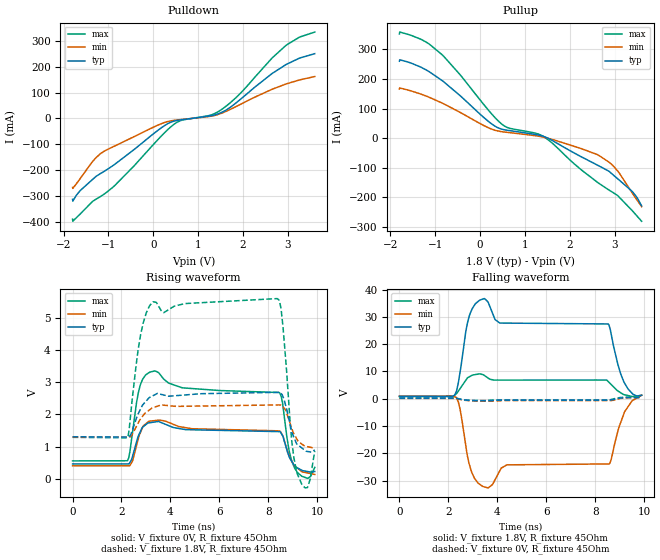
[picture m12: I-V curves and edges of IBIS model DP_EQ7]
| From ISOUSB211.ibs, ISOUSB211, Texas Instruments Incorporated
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[Model]   DP_EQ7
Model_type   Output
Polarity   Non-Inverting
Vmeas = 0.2
Vref = 0
Cref = 15pF
Rref = 45
|   typ   min   max
C_comp   5pF   3pF   8pF
[Voltage Range]   1.8   1.71   1.89
[Temperature Range]   27   150   -40
[Pullup Reference]   1.8   1.71   1.89
[Pulldown Reference]   0   0   0
[Power Clamp Reference]   1.8   1.71   1.89
[GND Clamp Reference]   0   0   0
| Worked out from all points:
|   slope of the pulldown table from 0 to 0.27 V, typ, clamps not added: 7.95 ohm
|   slope of the pullup table from 0 to 0.27 V, typ, clamps not added: 7.94 ohm
|   falling waveform, V_fixture 1.8V, R_fixture 45Ohm: 20-80 % time 71.7ps typ, 40.9ps min, 34.1ps max; typ from 0.895 V to 1.3 V
|   rising waveform, V_fixture 0V, R_fixture 45Ohm: 20-80 % time 286ps typ, 394ps min, 61.1ps max; typ from 0.46 V to 0.225 V
|   rising waveform, V_fixture 1.8V, R_fixture 45Ohm: 20-80 % time 252ps typ, 310ps min, 40.9ps max; typ from 1.3 V to 0.895 V
|   falling waveform, V_fixture 0V, R_fixture 45Ohm: 20-80 % time 184ps typ, 235ps min, 124ps max; typ from 0.225 V to 0.46 V
[Pulldown]
|   Voltage   I(typ)   I(min)   I(max)
-1.8V     -312.3mA   -266.2mA   -388.8mA
-1.795V   -319mA     -269.8mA   -396.8mA
-1.633V   -278.9mA   -232.8mA   -369.2mA
-1.179V   -212.7mA   -136mA     -301.6mA
-865.8mV  -177.8mA   -106.8mA   -260mA
73.8mV    -49.63mA   -27.98mA   -87.09mA
538.2mV   -7.266mA   -5.626mA   -13.71mA
1.294V    10.85mA    9.019mA    13.98mA
1.521V    23.18mA    20.15mA    34.45mA
1.899V    67.71mA    50.57mA    89.7mA
2.947V    206.8mA    132.3mA    280.4mA
3.6V      250.2mA    161.9mA    333.6mA
[Pullup]
|   Voltage   I(typ)   I(min)   I(max)
-1.8V     259.8mA    166.3mA    352.1mA
-1.795V   264.8mA    169.7mA    358.5mA
-1.325V   240.1mA    149.1mA    334.3mA
-849.6mV  194.9mA    118.9mA    282mA
381.6mV   36.3mA     24.84mA    61.51mA
613.8mV   26.64mA    19.55mA    35.63mA
1.402V    6.733mA    3.773mA    6.537mA
2.612V    -90.76mA   -55.24mA   -148.5mA
2.876V    -112.3mA   -81.28mA   -175.5mA
3.065V    -136.9mA   -110.7mA   -193.6mA
3.4V      -181.3mA   -187.3mA   -246.2mA
3.6V      -228.6mA   -231.2mA   -280.5mA
[Ramp]
R_load = 45
|   typ   min   max
dV/dt_r   0.140808/2.64432e-10   0.160407/3.48337e-10   0.120509/6.22032e-11
dV/dt_f   0.243789/4.77414e-11  0.210518/7.09993e-11   0.256824/2.36305e-09
[Falling Waveform]
V_fixture = 1.8V
V_fixture_min = 1.71V
V_fixture_max = 1.89V
R_fixture = 45Ohm
C_fixture = 0F
|   Time   V(typ)   V(min)   V(max)
0s        895mV      947.6mV    856.5mV
2.257ns   1.255V     713.3mV    1.343V
2.476ns   9.653V     -3.712V    3.69V
2.855ns   30.31V     -23.96V    8.039V
3.46ns    36.69V     -32.24V    8.615V
3.806ns   31.3V      -31.38V    6.957V
4.105ns   27.73V     -26.32V    6.853V
8.533ns   27.4V      -23.87V    6.319V
9.166ns   6.353V     -5.673V    1.535V
9.9ns     1.301V     1.298V     1.285V
[Rising Waveform]
V_fixture = 0V
V_fixture_min = 0V
V_fixture_max = 0V
R_fixture = 45Ohm
C_fixture = 0F
|   Time   V(typ)   V(min)   V(max)
0s        459.5mV    400.3mV    553.4mV
2.245ns   459.5mV    402.3mV    558.4mV
2.761ns   1.448V     1.411V     2.887V
3.359ns   1.76V      1.803V     3.343V
4.462ns   1.544V     1.604V     2.826V
8.444ns   1.462V     1.486V     2.675V
8.85ns    692mV      709.9mV    876.5mV
9.059ns   419.8mV    415mV      358.5mV
9.607ns   223.6mV    178.4mV    12.81mV
9.9ns     224.9mV    133mV      352.5mV
[Rising Waveform]
V_fixture = 1.8V
V_fixture_min = 1.71V
V_fixture_max = 1.89V
R_fixture = 45Ohm
C_fixture = 0F
|   Time   V(typ)   V(min)   V(max)
0s        1.301V     1.298V     1.285V
2.245ns   1.292V     1.295V     1.27V
2.776ns   2.156V     1.853V     4.442V
3.277ns   2.572V     2.202V     5.484V
8.356ns   2.679V     2.29V      5.587V
8.523ns   2.645V     2.285V     5.271V
8.96ns    1.458V     1.563V     1.169V
9.15ns    1.099V     1.255V     254.9mV
9.59ns    847.5mV    996.6mV    -277.8mV
9.9ns     895mV      947.6mV    856.5mV
[Falling Waveform]
|Gnd
V_fixture = 0V
V_fixture_min = 0V
V_fixture_max = 0V
R_fixture = 45Ohm
C_fixture = 0F
|   Time   V(typ)   V(min)   V(max)
0s        224.9mV    133mV      352.5mV
2.213ns   229.4mV    133mV      354.1mV
2.719ns   -488.5mV   -594mV     -486.9mV
3.39ns    -699.6mV   -854.6mV   -687.1mV
3.723ns   -679.2mV   -887.9mV   -518.7mV
4.393ns   -512.2mV   -642.5mV   -471.4mV
8.608ns   -505.3mV   -686.1mV   -371.7mV
8.914ns   68.88mV    -142.7mV   304.6mV
9.086ns   304.6mV    188.2mV    502.6mV
9.9ns     459.5mV    400.3mV    553.4mV
